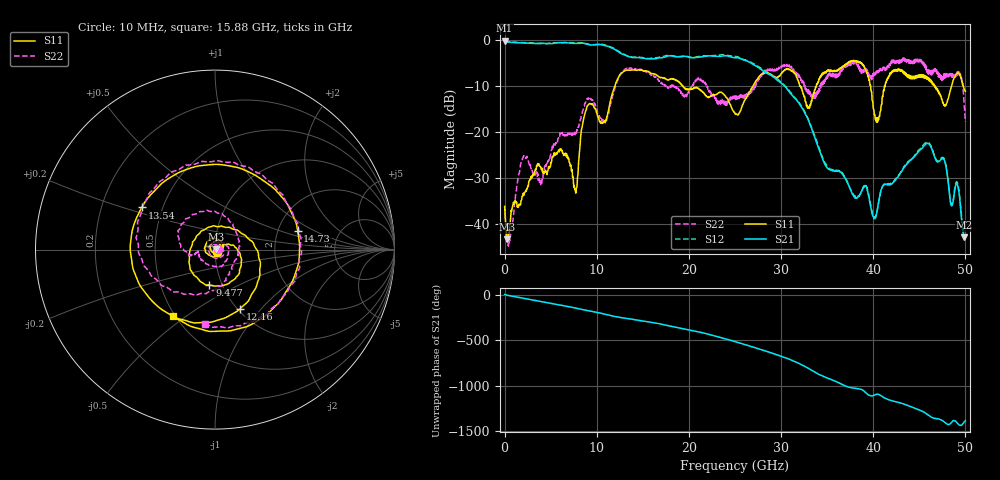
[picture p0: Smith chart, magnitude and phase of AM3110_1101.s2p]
# Hz S DB R 50.0
!freq dBS11 angS11 dBS21 angS21 dBS12 angS12 dBS22 angS22
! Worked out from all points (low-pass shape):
!   1601 points, 10 MHz to 50 GHz, reference 50 ohm
!   highest |S21| = -0.13 dB at 10 MHz (marker M1); lowest = -42.8 dB at 49.88 GHz (marker M2)
!   |S21| within 3 dB of the highest: start of sweep to 12.92 GHz
!   lowest |S11| = -43.3 dB at 322.4 MHz (marker M3), VSWR 1.01, Z = 50.6 + j0.241 ohm
!   |S11| at or under -10 dB: start of sweep to 11.97 GHz; 19.32 GHz to 26.95 GHz (7.636 GHz wide, 33 % of centre); 46.73 GHz to 48.5 GHz (1.774 GHz wide, 3.73 % of centre)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
!   |S22| runs from -44.8 to -3.9 dB; largest |S21 - S12| = 0.027
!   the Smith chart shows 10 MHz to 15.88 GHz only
!   S11 on the Smith chart (normalised r, x): 10 MHz: 1.02, -0.02; 9.477 GHz: 0.87, -0.36; 12.16 GHz: 1.03, -0.78; 13.54 GHz: 0.38, +0.23; 14.73 GHz: 2.57, +0.70; 15.88 GHz: 0.49, -0.45
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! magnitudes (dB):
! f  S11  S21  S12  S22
! 10 MHz  -36.2  -0.1  -0.1  -35.9
! 322.4 MHz  -43.3  -0.4  -0.3  -43.7
! 1.978 GHz  -33.8  -0.6  -0.5  -25.7
! 3.915 GHz  -27.6  -0.7  -0.7  -31.5
! 6.009 GHz  -23.6  -0.5  -0.6  -20.4
! 7.727 GHz  -33.2  -0.7  -0.6  -20.0
! 8.352 GHz  -19.4  -0.7  -0.6  -16.3
! 9.477 GHz  -14.0  -1.1  -1.0  -13.0
! 12.16 GHz  -8.9  -2.3  -2.1  -9.3
! 13.54 GHz  -6.5  -3.6  -3.6  -6.1
! 14.73 GHz  -6.5  -3.8  -3.7  -6.3
! 15.88 GHz  -7.2  -4.0  -3.9  -7.6
! 16.69 GHz  -7.9  -3.9  -3.7  -8.7
! 25 GHz  -16.0  -3.8  -3.5  -12.4
! 28.29 GHz  -7.0  -7.0  -6.7  -6.7
! 33.35 GHz  -13.3  -19.3  -19.1  -12.5
! 38.13 GHz  -4.5  -34.4  -34.0  -4.7
! 40.1 GHz  -15.7  -38.7  -38.5  -7.1
! 41.69 GHz  -7.9  -31.4  -31.2  -6.0
! 46 GHz  -8.2  -22.5  -22.3  -6.7
! 49.88 GHz  -10.6  -42.8  -41.7  -14.3
! 50 GHz  -11.1  -42.6  -41.4  -17.8
